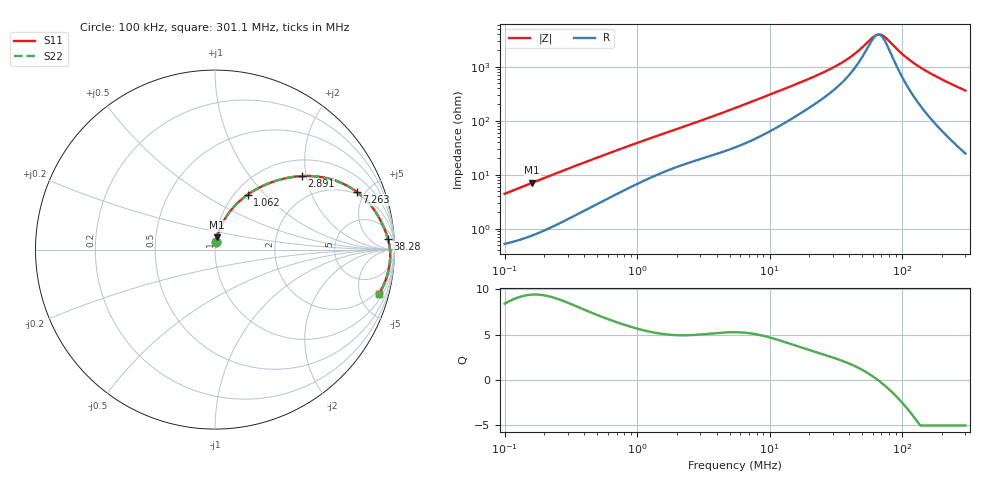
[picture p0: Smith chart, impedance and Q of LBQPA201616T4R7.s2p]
! LBQPA201616T4R7  S-PARAMETER MODEL  ( General Type )
! Model Generated by TAIYO YUDEN Corporation (http://www.ty-top.com)
! Version 1.0
! TAIYO YUDEN Control No. 191025NI43SB-FBB
! Copyright(c) 2019 TAIYO YUDEN CO.,LTD. All Rights Reserved.
! Product Description (link to TY-COMPAS)
! https://ds.yuden.co.jp/TYCOMPAS/or/detail?pn=LBQPA201616T4R7M&u=M
! Products Name : Inductors
! Characteristics :
!  Inductance : 4.7 uH , SRF(min) : 45 MHz , DC Resistance(max) : 0.481 Ohm
!  Rated Current : Saturation :550 mA , Temp Rise : 460 mA (20 degC)
!  Case Size : 2.0 x 1.6 / 0.079 x 0.063 [mm/inch] , Thickness : 1.6 / 0.063 [mm/inch]
!  (Conditions: Temperature = 25 degC , DC Bias Current/Voltage = 0A / 0V)
! External Node Assignments :
!  1  o---GGG---o  2
! GND o---------o GND
! Frequency Range : 0.1MHz  -  301.082333MHz  [ 402 STEP ]
# MHz S RI R 50
! Freq[MHz].  S11 Real  S11 Imag  S21 Real  S21 Imag  S12 Real  S12 Imag  S22 Real  S22 Imag
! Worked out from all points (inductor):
!   401 points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, 100 kHz to 301.1 MHz, reference 50 ohm
!   read as one part in series: L = 6.94 uH near 104.1 kHz
!   highest Q = 9.41 at 161.7 kHz (marker M1), where L = 6.91 uH
!   self-resonance near 65.8 MHz
!   S11 on the Smith chart (normalised r, x): 100 kHz: 1.01, +0.09; 1.062 MHz: 1.14, +0.80; 2.891 MHz: 1.38, +1.88; 7.263 MHz: 1.85, +4.36; 38.28 MHz: 13, +24; 301.1 MHz: 1.49, -7.20
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0.1  0.00706 0.0432  0.9929 -0.0432  0.9929 -0.0432  0.00706 0.0432
0.161704  0.0122 0.0688  0.9878 -0.0688  0.9878 -0.0688  0.0122 0.0688
0.382543  0.0434 0.1498  0.9566 -0.1498  0.9566 -0.1498  0.0434 0.1498
0.656888  0.096 0.2276  0.904 -0.2276  0.904 -0.2276  0.096 0.2276
1.062214  0.1814 0.3058  0.8186 -0.3058  0.8186 -0.3058  0.1814 0.3058
1.463388  0.2617 0.3528  0.7383 -0.3528  0.7383 -0.3528  0.2617 0.3528
2.890998  0.4824 0.4095  0.5176 -0.4095  0.5176 -0.4095  0.4824 0.4095
5.487097  0.7102 0.3685  0.2898 -0.3685  0.2898 -0.3685  0.7102 0.3685
7.262675  0.7901 0.3213  0.2099 -0.3213  0.2099 -0.3213  0.7901 0.3213
11.74405  0.8812 0.2292  0.1188 -0.2292  0.1188 -0.2292  0.8812 0.2292
20.99048  0.9354 0.1351  0.0646 -0.1351  0.0646 -0.1351  0.9354 0.1351
29.50303  0.9532 0.0914  0.0468 -0.0914  0.0468 -0.0914  0.9532 0.0914
38.27576  0.9631 0.0612  0.0369 -0.0612  0.0369 -0.0612  0.9631 0.0612
46.76177  0.9689 0.0387  0.0311 -0.0387  0.0311 -0.0387  0.9689 0.0387
59.46364  0.9738 0.0116  0.0262 -0.0116  0.0262 -0.0116  0.9738 0.0116
64.42262  0.9749 0.00245  0.0251 -0.00245  0.0251 -0.00245  0.9749 0.00245
71.20687  0.9759 -0.00922  0.0241 0.00922  0.0241 0.00922  0.9759 -0.00922
80.29753  0.9765 -0.0236  0.0235 0.0236  0.0235 0.0236  0.9765 -0.0236
104.174  0.9757 -0.0567  0.0243 0.0567  0.0243 0.0567  0.9757 -0.0567
135.1502  0.9711 -0.0938  0.0289 0.0938  0.0289 0.0938  0.9711 -0.0938
197.7217  0.9548 -0.1584  0.0452 0.1584  0.0452 0.1584  0.9548 -0.1584
301.0823  0.9141 -0.2482  0.0859 0.2482  0.0859 0.2482  0.9141 -0.2482
